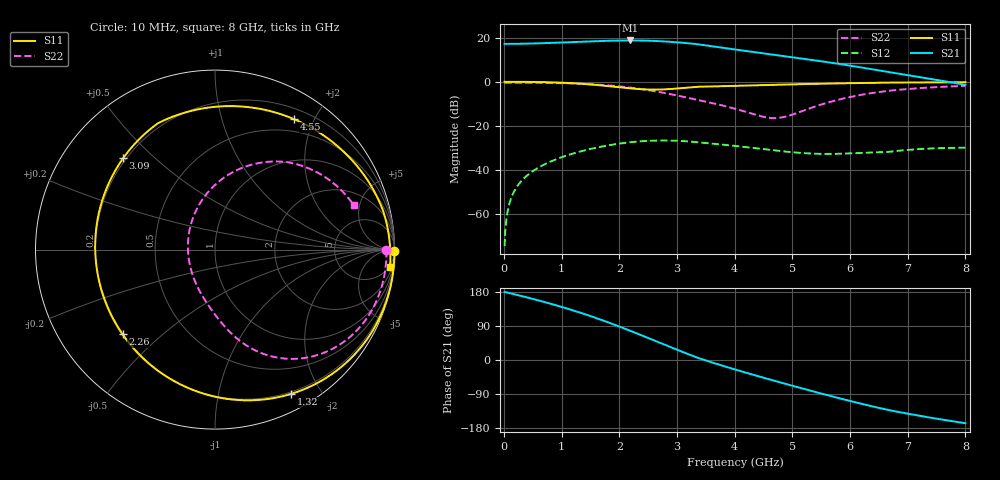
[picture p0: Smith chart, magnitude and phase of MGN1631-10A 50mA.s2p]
! Port[1] = GATE
! Port[2] = DRAIN
! [Type]  S-parameter s2p file touchstone ver. 1.0
! [Object]  MGN1631-10A
! [Bias]  50 mA
! [Version]  1.0
! [Date]  Thu May 19 10:13:03 2026
! [Source]  This file was created in JSC "ICC Milandr".
! [Disclaimer] Property of JSC "ICC Milandr". Unauthorized reproduction and/or distribution is strictly prohibited.
!  The file and the data are provided "AS IS" and with all faults and disclaim all warranties, express and implied, including
!  without limitation any implied warranties of merchantability, fitness for a particular purpose.
!  JSC "ICC Milandr" assumes no liability for:
!  1) the accuracy of the data provided;
!  2) the proper functioning of this data;
!  3) infringement of patents, copyrights or intellectual property rights resulting from the use of this data.
!  JSC "ICC Milandr" reserves the right to make changes to the products and the data without prior notice.
!  Please, be aware that your receipt and use of the file provided shall serve as acceptance of these terms and conditions.
!  If you do not accept these terms, you should return or destroy this file and any other accompanying information immediately.
# Hz S MA R 12.5
! freq  S11mag  S11ang  S21mag  S21ang  S12mag  S12ang  S22mag  S22ang
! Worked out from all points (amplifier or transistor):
!   800 points, 10 MHz to 8 GHz, reference 12.5 ohm
!   highest |S21| = 18.8 dB at 2.19 GHz (marker M1)
!   |S21| within 3 dB of that: start of sweep to 3.704 GHz
!   unconditionally stable (mu >= 1): 4.494 GHz to 5.865 GHz
!   at 1.34 GHz: K = 0.31, MSG = 24.8 dB, |S12| = -31.5 dB
!   at 4.01 GHz: K = 0.86, MSG = 21.9 dB, |S12| = -29.0 dB
!   at 8 GHz: K = 0.43, MSG = 14.3 dB, |S12| = -29.8 dB
!   S11 on the Smith chart (normalised r, x): 10 MHz: open; 1.32 GHz: 0.18, -1.64; 2.26 GHz: 0.20, -0.37; 3.09 GHz: 0.19, +0.40; 4.55 GHz: 0.33, +1.72; 8 GHz: 4, -19
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1e7  1 -0.4  7.254 179.5  0.0001883 85.6  0.9555 -0.2
9e7  1 -3.7  7.248 176.7  0.001682 86.8  0.9558 -1.9
2e8  1 -8.2  7.269 172.7  0.003745 83.7  0.9558 -4.3
7.4e8  0.9816 -31.7  7.567 151.4  0.01424 66.0  0.9465 -16.2
1.04e9  0.9521 -46.5  7.83 138.2  0.02041 54.9  0.9309 -23.4
1.32e9  0.9088 -62.2  8.105 124.9  0.02632 43.5  0.9061 -30.6
1.35e9  0.9033 -64.0  8.134 123.4  0.02696 42.2  0.9027 -31.4
1.81e9  0.7999 -96.2  8.534 99.1  0.03637 21.2  0.8311 -44.1
2.19e9  0.7111 -130.4  8.672 77.0  0.04272 1.9  0.7407 -55.3
2.26e9  0.6981 -137.5  8.666 72.8  0.04364 -1.8  0.7212 -57.3
2.46e9  0.6725 -158.9  8.584 60.5  0.04566 -12.6  0.6616 -63.2
2.68e9  0.6684 176.9  8.377 46.9  0.04675 -24.6  0.5919 -69.3
2.89e9  0.688 154.5  8.072 33.8  0.04662 -36.1  0.5249 -74.9
3.09e9  0.7218 135.1  7.703 21.6  0.04549 -46.8  0.4638 -80.0
3.31e9  0.7665 116.5  7.237 8.6  0.04327 -58.2  0.4018 -85.7
3.52e9  0.7812 102.8  6.638 -2.2  0.04092 -65.7  0.3512 -91.3
4.01e9  0.8129 78.3  5.407 -25.2  0.03529 -77.3  0.2445 -110.9
4.55e9  0.8496 58.9  4.351 -48.9  0.02931 -82.1  0.1561 -158.6
5.34e9  0.898 38.4  3.145 -82.0  0.02364 -73.7  0.2611 110.5
5.97e9  0.9314 25.4  2.363 -107.0  0.02379 -62.2  0.444 76.8
6.67e9  0.961 13.0  1.665 -132.2  0.02584 -57.0  0.6269 51.2
8e9  0.9801 -5.7  0.8616 -166.8  0.0322 -78.6  0.8112 17.9
